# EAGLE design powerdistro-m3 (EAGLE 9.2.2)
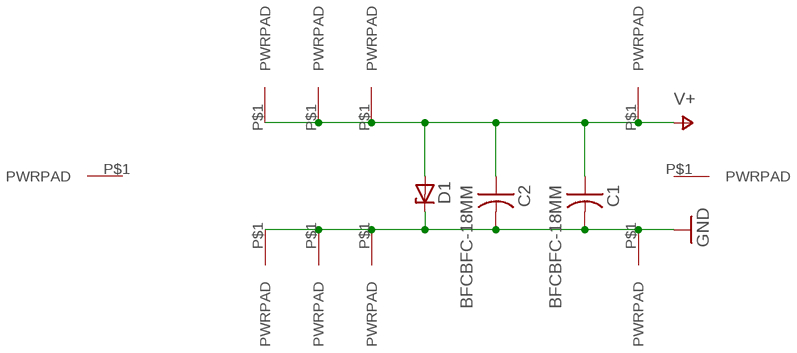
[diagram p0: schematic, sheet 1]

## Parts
C1  BFCBFC-18MM  [BFC-18MM-7-5MM]
C2  BFCBFC-18MM  [BFC-18MM-7-5MM]
D1  ZENER_DIODE  [SMA-DO-214AC]
J1  PWRPADM3-STANDOFF  [PWRPAD_M3_STANDOFF]
J2  PWRPADM3-STANDOFF  [PWRPAD_M3_STANDOFF]
J3  PWRPADM3-STANDOFF  [PWRPAD_M3_STANDOFF]
J4  PWRPADM3-STANDOFF  [PWRPAD_M3_STANDOFF]
J5  PWRPADM3-STANDOFF  [PWRPAD_M3_STANDOFF]
J6  PWRPADM3-STANDOFF  [PWRPAD_M3_STANDOFF]
J7  PWRPADM3-STANDOFF  [PWRPAD_M3_STANDOFF]
J8  PWRPADM3-STANDOFF  [PWRPAD_M3_STANDOFF]
J11  PWRPADM3-STANDOFF  [PWRPAD_M3_STANDOFF]
J12  PWRPADM3-STANDOFF  [PWRPAD_M3_STANDOFF]

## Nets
GND: C1.P$1 C2.P$1 D1.P$2(CATHODE) J2.P$1(PWRPAD) J6.P$1(PWRPAD) J7.P$1(PWRPAD) J8.P$1(PWRPAD)
V+: C1.P$2 C2.P$2 D1.P$1(ANODE) J1.P$1(PWRPAD) J3.P$1(PWRPAD) J4.P$1(PWRPAD) J5.P$1(PWRPAD)
Unconnected: J11.P$1(PWRPAD) J12.P$1(PWRPAD)

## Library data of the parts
C1 C2 = power:BFC
D1 = passives:ZENER_DIODE: zener diode
J1-J8 J11 J12 = power:PWRPAD

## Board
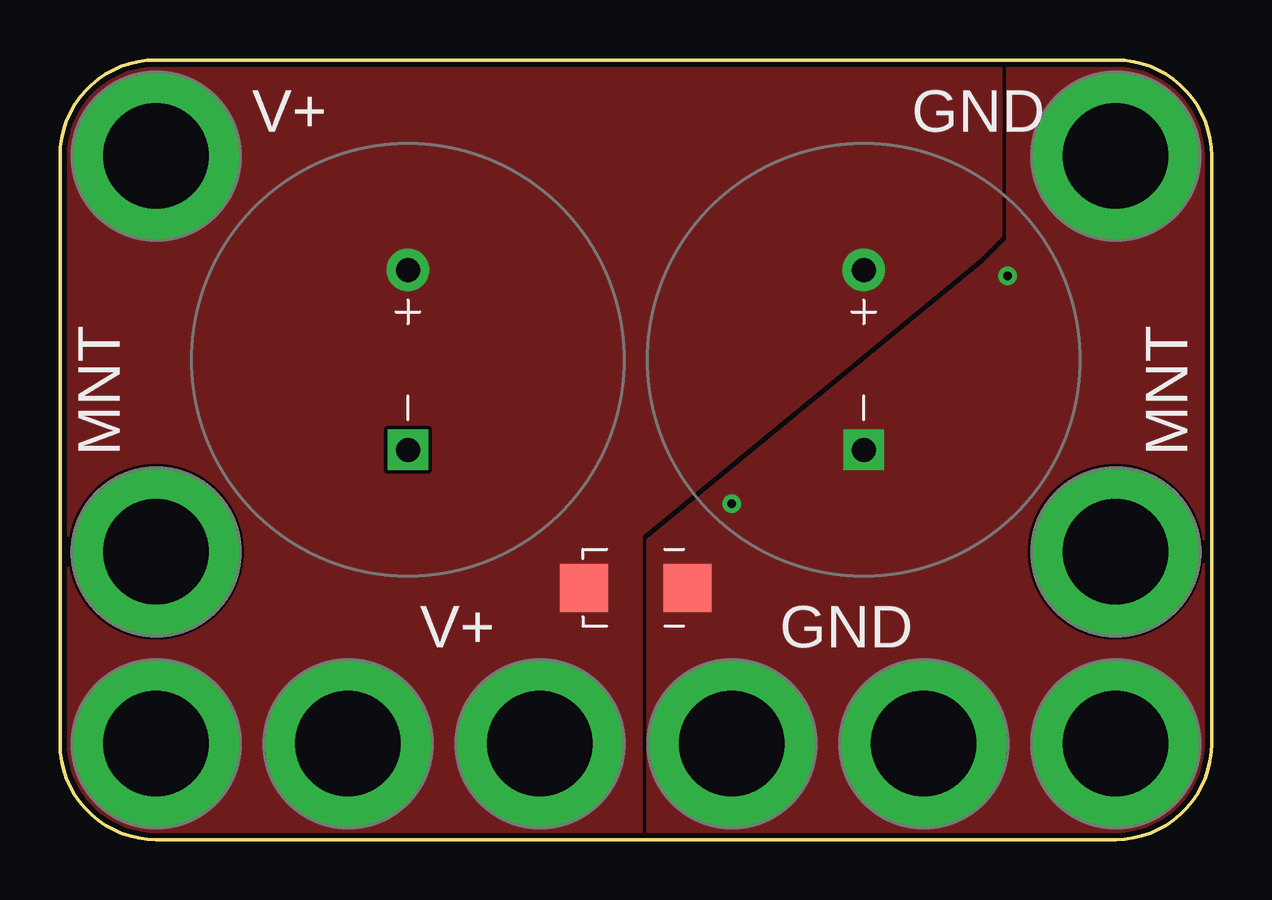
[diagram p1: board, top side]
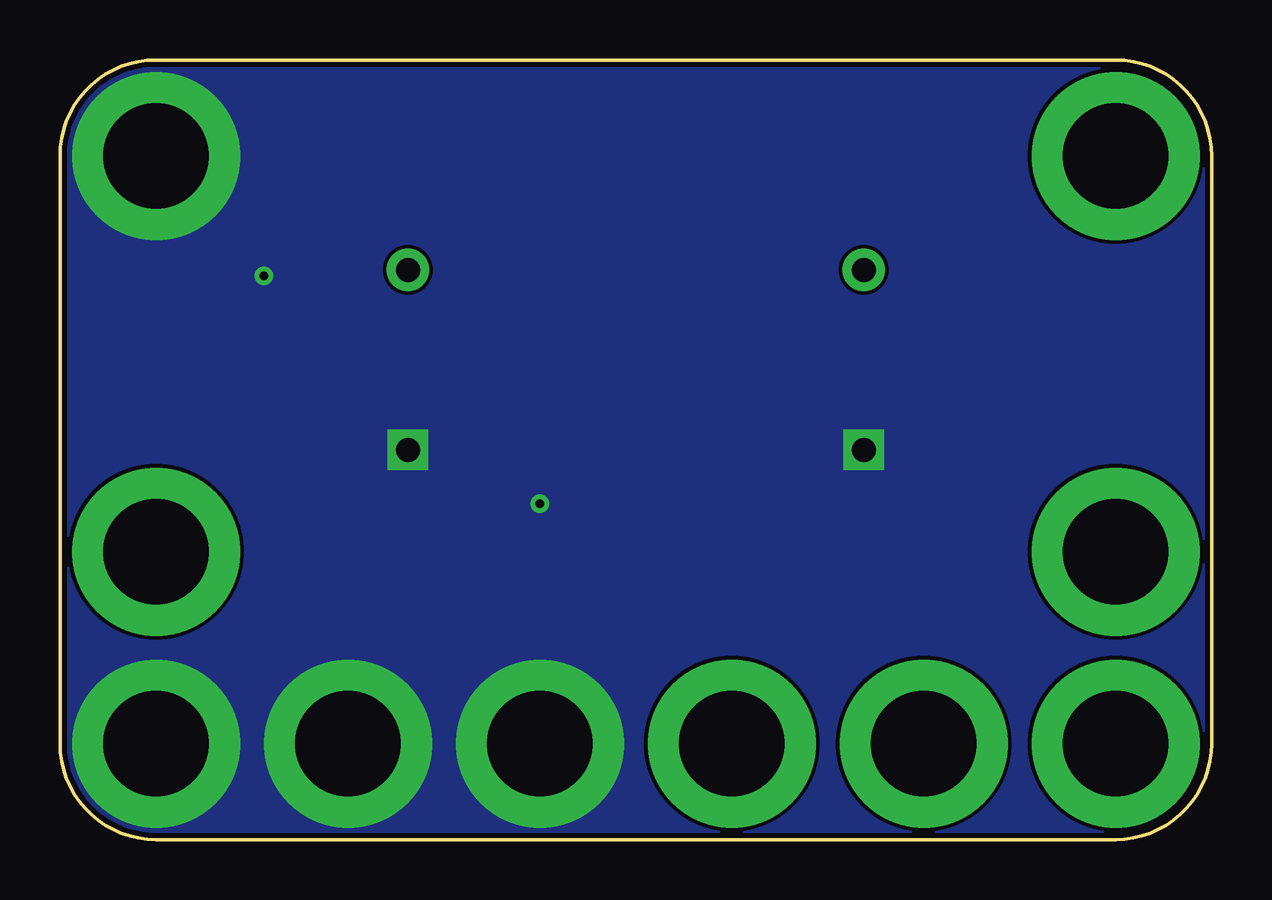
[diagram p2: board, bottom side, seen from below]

Size 48 x 32.5 mm. Coordinates in mm from the lower left corner, seen from the top.
Outline: 0,4 0,28.5 arc-90 4,32.5 44,32.5 arc-90 48,28.5 48,4 arc-90 44,0 4,0 arc-90 0,4
Copper layers (1*16): Top 0.035mm / dielectric 1.5mm / Bottom 0.035mm
Design rules "default *": minimum track width 6mil, minimum drill 0.35mm, track to track 6mil, track to pad 6mil, pad to pad 6mil, via to via 6mil, smd to smd 6mil, copper to edge 8mil, drill to drill 6mil, minimum pad ring 10mil, minimum via ring 8mil, stop-mask expansion 4mil, vias tented up to drill 0mil, thermal gap 10mil

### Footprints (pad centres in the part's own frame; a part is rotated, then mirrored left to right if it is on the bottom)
BFC-18MM-7-5MM = drill 1 pad 1.676 square: P$1 -3.75,0 | drill 1 pad 1.778: P$2 3.75,0
SMA-DO-214AC = smd 2 x 2: P$1 -2.15,0; P$2 2.15,0
PWRPAD_M3_STANDOFF = drill 4.4 pad 7: P$1 0,0

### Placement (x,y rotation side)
C1  14.5,20 90 top
C2  33.5,20 90 top
D1  24,10.5 0 top
J1  4,4 0 top
J2  36,4 0 top
J3  20,4 0 top
J4  12,4 0 top
J5  4,28.5 0 top
J6  44,28.5 0 top
J7  44,4 0 top
J8  28,4 0 top
J11  4,12 0 top
J12  44,12 0 top

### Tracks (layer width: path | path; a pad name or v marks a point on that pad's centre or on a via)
GND  (via drill 0.35)
  other vias: 28,14 39.5,23.5
  pour Bottom (no thermals): -1.5,33.5 49,33.5 49,-1 -1.5,-1
  pour Top (no thermals): 24.5,12 24.5,-2.5 51,-2.5 51,12.5 51,35 40,35 39.5,34.5 39.5,25 38.5,24 24.5,12.5
V+
  pour Top (rank 3, no thermals): -0.5,33 48.5,33 48.5,-0.5 -1,-0.5 -1,33

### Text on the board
tPlace: V+ | GND | MNT | MNT | V+ | GND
